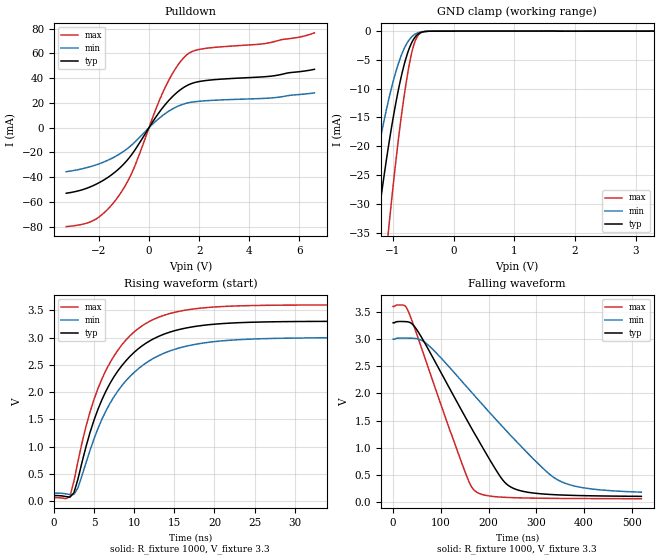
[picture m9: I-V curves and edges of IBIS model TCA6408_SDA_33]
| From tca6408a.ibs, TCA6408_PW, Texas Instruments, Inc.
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[Model]   TCA6408_SDA_33
Model_type  I/O_open_drain
Vinl=0.9
Vinh=2.52
Enable   Active-Low
Vref =   3.3
Rref =   1000
Cref =   50p
Vmeas =   1.65
| variable   typ   min   max
C_comp   3.09pF   2.15pF   3.49pF
| C_pulldown   1.93pF   0.79pF   2.61pF
| C_tri-state   3.09pF   2.15pF   3.49pF
[Temperature Range]   40   100   -40
| Ambient temperature   25   85   -40
[Voltage range]   3.3   3   3.6
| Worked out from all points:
|   slope of the pulldown table from 0 to 0.495 V, typ, clamps not added: 33.5 ohm
|   GND clamp passes 1 mA (typ) near -0.63 V on its own axis
|   rising waveform, R_fixture 1000, V_fixture 3.3: 20-80 % time 5.95ns typ, 6.49ns min, 5.55ns max; typ from 0.099 V to 3.3 V
|   falling waveform, R_fixture 1000, V_fixture 3.3: 20-80 % time 122ns typ, 177ns min, 84.5ns max; typ from 3.3 V to 0.106 V
[GND Clamp]
| TCA6408_SDA_33
|   Voltage   I(typ)   I(min)   I(max)
-3.3V     -264.3mA   -197.2mA   -365.9mA
-1.46V    -51.45mA   -34.2mA    -81.86mA
-1.26V    -34.06mA   -21.77mA   -56.25mA
-1.075V   -20.22mA   -12.19mA   -35.04mA
-1.06V    -19.22mA   -11.51mA   -33.46mA
-940mV    -11.89mA   -6.708mA   -21.65mA
-815mV    -5.903mA   -3.074mA   -11.38mA
-710mV    -2.491mA   -1.239mA   -4.787mA
-615mV    -804.7uA   -423.4uA   -1.293mA
-540mV    -241.7uA   -151uA     -300.8uA
-405mV    -18.25uA   -15.19uA   -16.16uA
3.3V      407.3pA    2.093uA    -3.305uA
[Pulldown]
| TCA6408_SDA_33
|   Voltage   I(typ)   I(min)   I(max)
-3.3V     -52.92mA   -35.52mA   -79.84mA
-2.15V    -46.04mA   -30.28mA   -74.19mA
-1.68V    -40.67mA   -26.63mA   -66.56mA
-1.215V   -33.45mA   -21.75mA   -55.31mA
-625mV    -19.9mA    -12.71mA   -33.86mA
255mV     8.017mA    4.951mA    14.05mA
670mV     19.21mA    11.72mA    33.54mA
1.115V    28.43mA    17.02mA    49.47mA
1.535V    34.24mA    19.97mA    59.3mA
2.105V    37.65mA    21.54mA    63.61mA
4.62V     41.17mA    23.71mA    67.96mA
6.6V      47.17mA    28.14mA    76.63mA
[Ramp]
| TCA6408_SDA_33
| variable   typ   min   max
dV/dt_r   1.94/5.95E-09   1.73/6.50E-09   2.14/5.54E-09
dV/dt_f   1.93/1.23E-07   1.70/1.78E-07   2.14/8.51E-08
R_load = 1000
[Rising Waveform]
| TCA6408_SDA_33
R_fixture =   1000
C_fixture =   0
L_fixture =   0
V_fixture =   3.3
V_fixture_min = 3
V_fixture_max = 3.6
|   Time   V(typ)   V(min)   V(max)
0s        98.69mV    143.4mV    61.66mV
2ns       70.39mV    119.2mV    81mV
2.5ns     149.4mV    119.9mV    363.5mV
4ns       994.5mV    697.6mV    1.365V
5.5ns     1.685V     1.332V     2.067V
7ns       2.16V      1.795V     2.541V
9ns       2.579V     2.212V     2.96V
14ns      3.078V     2.73V      3.423V
21.5ns    3.262V     2.947V     3.574V
520ns     3.3V       3V         3.6V
[Falling Waveform]
| TCA6408_SDA_33
R_fixture =   1000
C_fixture =   0
L_fixture =   0
V_fixture =   3.3
V_fixture_min = 3
V_fixture_max = 3.6
|   Time   V(typ)   V(min)   V(max)
0s        3.3V       3V         3.6V
22ns      3.322V     3.018V     3.622V
31.5ns    3.315V     3.017V     3.517V
73.5ns    2.815V     2.889V     2.475V
152ns     1.553V     2.143V     528.1mV
172.5ns   1.233V     1.94V      199.5mV
228ns     426mV      1.399V     91.23mV
257ns     235.8mV    1.128V     80.31mV
356.5ns   129.7mV    360.2mV    67.54mV
520ns     106.4mV    182.9mV    63.03mV
